|   stm32f401_d_e_uqfn48 IBIS Model
[IBIS ver]   4.2
[File name]  stm32f401_d_e_uqfn48.ibs
[File Rev]   1.0
[Date]   09-06-2015
[Source] Data Created at STMicroelectronics
[Notes]   File originated from ELDO simulations.
[Disclaimer]  This information is for modeling purpose only and is
   not guaranted. The information is subject to change without
   notice.
[Copyright] Copyright 2015 STMicroelectronics Inc.
[Component] stm32f401_d_e_uqfn48
[Manufacturer] STMicroelectronics
[Package]
| variable   typ   min   max
R_pkg   0.0   NA   NA
L_pkg   0.0H   NA   NA
C_pkg   0.0F   NA   NA
[Pin]   signal_name   model_name   R_pin   L_pin   C_pin
1 VBAT POWER 0.053 3.42534E-09 9.041E-14
2 PC13-ANTI_TAMP io8p_arwsudq_ft_v33 0.048377332 2.91404E-09 6.443E-14
3 PC14-OSC32_IN io8p_arwsudq_ft 0.044678997 2.50442E-09 4.365E-14
4 PC15-OSC32_OUT io8p_arsudq_ft 0.041905328 2.19704E-09 2.807E-14
5 PH0-OSC_IN io8p_arsudq_ft 0.040056325 1.9919E-09 1.769E-14
6 PH1-OSC_OUT io8p_arsudq_ft 0.03913 1.89021E-09 1.24625E-14
7 NRST ioreset_ft_v33 0.03913 1.89021E-09 1.24625E-14
8 VSSA GND 0.040057312 1.98992E-09 1.775E-14
9 VDDA POWER 0.041906973 2.19374E-09 2.817E-14
10 PA0-WKUP io8p_arwsudq_ft_v33 0.0446813 2.4998E-09 4.379E-14
11 PA1 io8p_arwsudq_ft 0.048380293 2.9081E-09 6.461E-14
12 PA2 io8p_arwsudq_ft 0.053 3.42534E-09 9.041E-14
13 PA3 io8p_arwsudq_ft 0.053 3.42534E-09 9.041E-14
14 PA4 io8p_ar3wsudq_ft 0.048377332 2.91404E-09 6.443E-14
15 PA5 io8p_ar3wsudq_ft 0.044678997 2.50442E-09 4.365E-14
16 PA6 io8p_ar3wsudq_ft 0.041905328 2.19704E-09 2.807E-14
17 PA7 io8p_arwsudq_ft 0.040056325 1.9919E-09 1.769E-14
18 PB0 io8p_ar3wsudq_ft 0.03913 1.89021E-09 1.24625E-14
19 PB1 io8p_ar3wsudq_ft 0.03913 1.89021E-09 1.24625E-14
20 PB2 io8p_arwsudq_ft 0.040057312 1.98992E-09 1.775E-14
21 PB10 io8p_arsudq_i2cin_ft 0.041906973 2.19374E-09 2.817E-14
22 VCAP1 POWER 0.0446813 2.4998E-09 4.379E-14
23 VSS GND 0.048380293 2.9081E-09 6.461E-14
24 VDD POWER 0.053 3.42534E-09 9.041E-14
25 PB12 io8p_arsudq_ft 0.053 3.42534E-09 9.041E-14
26 PB13 io8p_arsudq_ft 0.048377332 2.91404E-09 6.443E-14
27 PB14 io8p_arsudq_ft 0.044678997 2.50442E-09 4.365E-14
28 PB15 io8p_arsudq_ft 0.041905328 2.19704E-09 2.807E-14
29 PA8 io8p_arsudq_i2cin_ft 0.040056325 1.9919E-09 1.769E-14
30 PA9 io8usb_vbus_otg_ft 0.03913 1.89021E-09 1.24625E-14
31 PA10 io8usb_id_otg_ft 0.03913 1.89021E-09 1.24625E-14
32 PA11 io8usb_lsfs_otg_ft 0.040057312 1.98992E-09 1.775E-14
33 PA12 io8usb_lsfs_otg_ft 0.041906973 2.19374E-09 2.817E-14
34 PA13 io8p_arsudq_ft 0.0446813 2.4998E-09 4.379E-14
35 VSS GND 0.048380293 2.9081E-09 6.461E-14
36 VDD POWER 0.053 3.42534E-09 9.041E-14
37 PA14 io8p_arsudq_ft 0.053 3.42534E-09 9.041E-14
38 PA15 io8p_arsudq_ft 0.048377332 2.91404E-09 6.443E-14
39 PB3 io8p_arsudq_i2cin_ft 0.044678997 2.50442E-09 4.365E-14
40 PB4 io8p_arsudq_i2cin_ft 0.041905328 2.19704E-09 2.807E-14
41 PB5 io8p_ar3wsudq_ft 0.040056325 1.9919E-09 1.769E-14
42 PB6 io8p_arsudq_i2cin_ft 0.03913 1.89021E-09 1.24625E-14
43 PB7 io8p_arsudq_i2cin_ft 0.03913 1.89021E-09 1.24625E-14
44 BOOT0 vpp_test_hv 0.040057312 1.98992E-09 1.775E-14
45 PB8 io8p_arsudq_i2cin_ft 0.041906973 2.19374E-09 2.817E-14
46 PB9 io8p_arsudq_i2cin_ft 0.0446813 2.4998E-09 4.379E-14
47 VSS GND 0.048380293 2.9081E-09 6.461E-14
48 VDD POWER 0.053 3.42534E-09 9.041E-14
[Diff Pin]   inv_pin   vdiff   tdelay_typ  tdelay_min  tdelay_max
32 33 200mV   NA   NA   NA
[Model Selector] io8p_ar3wsudq_ft
io8p00_ar3wsudq_ft_pd_lv  "SPEED00 1P8V, PD=40kOhm"
io8p00_ar3wsudq_ft_pu_lv  "SPEED00 1P8V, PU=40kOhm"
io8p00_ar3wsudq_ft_lv  "SPEED00 1P8V"
io8p01_ar3wsudq_ft_pd_lv  "SPEED01 1P8V, PD=40kOhm"
io8p01_ar3wsudq_ft_pu_lv  "SPEED01 1P8V, PU=40kOhm"
io8p01_ar3wsudq_ft_lv  "SPEED01 1P8V"
io8p10_ar3wsudq_ft_pd_lv  "SPEED10 1P8V, PD=40kOhm"
io8p10_ar3wsudq_ft_pu_lv  "SPEED10 1P8V, PU=40kOhm"
io8p10_ar3wsudq_ft_lv  "SPEED10 1P8V"
io8p11_ar3wsudq_ft_pd_lv  "SPEED11 1P8V, PD=40kOhm"
io8p11_ar3wsudq_ft_pu_lv  "SPEED11 1P8V, PU=40kOhm"
io8p11_ar3wsudq_ft_lv  "SPEED11 1P8V"
io8p00_ar3wsudq_ft_pd  "SPEED00, PD=40kOhm"
io8p00_ar3wsudq_ft_pu  "SPEED00, PU=40kOhm"
io8p00_ar3wsudq_ft  "SPEED00"
io8p01_ar3wsudq_ft_pd  "SPEED01, PD=40kOhm"
io8p01_ar3wsudq_ft_pu  "SPEED01, PU=40kOhm"
io8p01_ar3wsudq_ft  "SPEED01"
io8p10_ar3wsudq_ft_pd  "SPEED10, PD=40kOhm"
io8p10_ar3wsudq_ft_pu  "SPEED10, PU=40kOhm"
io8p10_ar3wsudq_ft  "SPEED10"
io8p11_ar3wsudq_ft_pd  "SPEED11, PD=40kOhm"
io8p11_ar3wsudq_ft_pu  "SPEED11, PU=40kOhm"
io8p11_ar3wsudq_ft  "SPEED11"
[Model Selector] io8p_arsudq_ft
io8p00_arsudq_ft_pd_lv  "SPEED00 1P8V, PD=40kOhm"
io8p00_arsudq_ft_pu_lv  "SPEED00 1P8V, PU=40kOhm"
io8p00_arsudq_ft_lv  "SPEED00 1P8V"
io8p01_arsudq_ft_pd_lv  "SPEED01 1P8V, PD=40kOhm"
io8p01_arsudq_ft_pu_lv  "SPEED01 1P8V, PU=40kOhm"
io8p01_arsudq_ft_lv  "SPEED01 1P8V"
io8p10_arsudq_ft_pd_lv  "SPEED10 1P8V, PD=40kOhm"
io8p10_arsudq_ft_pu_lv  "SPEED10 1P8V, PU=40kOhm"
io8p10_arsudq_ft_lv  "SPEED10 1P8V"
io8p11_arsudq_ft_pd_lv  "SPEED11 1P8V, PD=40kOhm"
io8p11_arsudq_ft_pu_lv  "SPEED11 1P8V, PU=40kOhm"
io8p11_arsudq_ft_lv  "SPEED11 1P8V"
io8p00_arsudq_ft_pd  "SPEED00, PD=40kOhm"
io8p00_arsudq_ft_pu  "SPEED00, PU=40kOhm"
io8p00_arsudq_ft  "SPEED00"
io8p01_arsudq_ft_pd  "SPEED01, PD=40kOhm"
io8p01_arsudq_ft_pu  "SPEED01, PU=40kOhm"
io8p01_arsudq_ft  "SPEED01"
io8p10_arsudq_ft_pd  "SPEED10, PD=40kOhm"
io8p10_arsudq_ft_pu  "SPEED10, PU=40kOhm"
io8p10_arsudq_ft  "SPEED10"
io8p11_arsudq_ft_pd  "SPEED11, PD=40kOhm"
io8p11_arsudq_ft_pu  "SPEED11, PU=40kOhm"
io8p11_arsudq_ft  "SPEED11"
[Model Selector] io8p_arsudq_i2cin_ft
io8p00_arsudq_i2cin_ft_pd_lv  "SPEED00 1P8V, PD=40kOhm"
io8p00_arsudq_i2cin_ft_pu_lv  "SPEED00 1P8V, PU=40kOhm"
io8p00_arsudq_i2cin_ft_lv  "SPEED00 1P8V"
io8p01_arsudq_i2cin_ft_pd_lv  "SPEED01 1P8V, PD=40kOhm"
io8p01_arsudq_i2cin_ft_pu_lv  "SPEED01 1P8V, PU=40kOhm"
io8p01_arsudq_i2cin_ft_lv  "SPEED01 1P8V"
io8p10_arsudq_i2cin_ft_pd_lv  "SPEED10 1P8V, PD=40kOhm"
io8p10_arsudq_i2cin_ft_pu_lv  "SPEED10 1P8V, PU=40kOhm"
io8p10_arsudq_i2cin_ft_lv  "SPEED10 1P8V"
io8p11_arsudq_i2cin_ft_pd_lv  "SPEED11 1P8V, PD=40kOhm"
io8p11_arsudq_i2cin_ft_pu_lv  "SPEED11 1P8V, PU=40kOhm"
io8p11_arsudq_i2cin_ft_lv  "SPEED11 1P8V"
io8p00_arsudq_i2cin_ft_pd  "SPEED00, PD=40kOhm"
io8p00_arsudq_i2cin_ft_pu  "SPEED00, PU=40kOhm"
io8p00_arsudq_i2cin_ft  "SPEED00"
io8p01_arsudq_i2cin_ft_pd  "SPEED01, PD=40kOhm"
io8p01_arsudq_i2cin_ft_pu  "SPEED01, PU=40kOhm"
io8p01_arsudq_i2cin_ft  "SPEED01"
io8p10_arsudq_i2cin_ft_pd  "SPEED10, PD=40kOhm"
io8p10_arsudq_i2cin_ft_pu  "SPEED10, PU=40kOhm"
io8p10_arsudq_i2cin_ft  "SPEED10"
io8p11_arsudq_i2cin_ft_pd  "SPEED11, PD=40kOhm"
io8p11_arsudq_i2cin_ft_pu  "SPEED11, PU=40kOhm"
io8p11_arsudq_i2cin_ft  "SPEED11"
[Model Selector] io8p_arwsudq_ft
io8p00_arwsudq_ft_pd_lv  "SPEED00 1P8V, PD=40kOhm"
io8p00_arwsudq_ft_pu_lv  "SPEED00 1P8V, PU=40kOhm"
io8p00_arwsudq_ft_lv  "SPEED00 1P8V"
io8p01_arwsudq_ft_pd_lv  "SPEED01 1P8V, PD=40kOhm"
io8p01_arwsudq_ft_pu_lv  "SPEED01 1P8V, PU=40kOhm"
io8p01_arwsudq_ft_lv  "SPEED01 1P8V"
io8p10_arwsudq_ft_pd_lv  "SPEED10 1P8V, PD=40kOhm"
io8p10_arwsudq_ft_pu_lv  "SPEED10 1P8V, PU=40kOhm"
io8p10_arwsudq_ft_lv  "SPEED10 1P8V"
io8p11_arwsudq_ft_pd_lv  "SPEED11 1P8V, PD=40kOhm"
io8p11_arwsudq_ft_pu_lv  "SPEED11 1P8V, PU=40kOhm"
io8p11_arwsudq_ft_lv  "SPEED11 1P8V"
io8p00_arwsudq_ft_pd  "SPEED00, PD=40kOhm"
io8p00_arwsudq_ft_pu  "SPEED00, PU=40kOhm"
io8p00_arwsudq_ft  "SPEED00"
io8p01_arwsudq_ft_pd  "SPEED01, PD=40kOhm"
io8p01_arwsudq_ft_pu  "SPEED01, PU=40kOhm"
io8p01_arwsudq_ft  "SPEED01"
io8p10_arwsudq_ft_pd  "SPEED10, PD=40kOhm"
io8p10_arwsudq_ft_pu  "SPEED10, PU=40kOhm"
io8p10_arwsudq_ft  "SPEED10"
io8p11_arwsudq_ft_pd  "SPEED11, PD=40kOhm"
io8p11_arwsudq_ft_pu  "SPEED11, PU=40kOhm"
io8p11_arwsudq_ft  "SPEED11"
[Model Selector] io8p_arwsudq_ft_v33
io8p00_arwsudq_ft_v33_pd_lv  "SPEED00 1P8V, PD=40kOhm"
io8p00_arwsudq_ft_v33_pu_lv  "SPEED00 1P8V, PU=40kOhm"
io8p00_arwsudq_ft_v33_lv  "SPEED00 1P8V"
io8p01_arwsudq_ft_v33_pd_lv  "SPEED01 1P8V, PD=40kOhm"
io8p01_arwsudq_ft_v33_pu_lv  "SPEED01 1P8V, PU=40kOhm"
io8p01_arwsudq_ft_v33_lv  "SPEED01 1P8V"
io8p10_arwsudq_ft_v33_pd_lv  "SPEED10 1P8V, PD=40kOhm"
io8p10_arwsudq_ft_v33_pu_lv  "SPEED10 1P8V, PU=40kOhm"
io8p10_arwsudq_ft_v33_lv  "SPEED10 1P8V"
io8p11_arwsudq_ft_v33_pd_lv  "SPEED11 1P8V, PD=40kOhm"
io8p11_arwsudq_ft_v33_pu_lv  "SPEED11 1P8V, PU=40kOhm"
io8p11_arwsudq_ft_v33_lv  "SPEED11 1P8V"
io8p00_arwsudq_ft_v33_pd  "SPEED00, PD=40kOhm"
io8p00_arwsudq_ft_v33_pu  "SPEED00, PU=40kOhm"
io8p00_arwsudq_ft_v33  "SPEED00"
io8p01_arwsudq_ft_v33_pd  "SPEED01, PD=40kOhm"
io8p01_arwsudq_ft_v33_pu  "SPEED01, PU=40kOhm"
io8p01_arwsudq_ft_v33  "SPEED01"
io8p10_arwsudq_ft_v33_pd  "SPEED10, PD=40kOhm"
io8p10_arwsudq_ft_v33_pu  "SPEED10, PU=40kOhm"
io8p10_arwsudq_ft_v33  "SPEED10"
io8p11_arwsudq_ft_v33_pd  "SPEED11, PD=40kOhm"
io8p11_arwsudq_ft_v33_pu  "SPEED11, PU=40kOhm"
io8p11_arwsudq_ft_v33  "SPEED11"
[Model Selector] io8usb_id_otg_ft
io8p00_id_otg_ft_pd_lv  "SPEED00 1P8V, PD=14kOhm"
io8p00_id_otg_ft_pu_lv  "SPEED00 1P8V, PU=14kOhm"
io8p00_id_otg_ft_lv  "SPEED00 1P8V"
io8p01_id_otg_ft_pd_lv  "SPEED01 1P8V, PD=14kOhm"
io8p01_id_otg_ft_pu_lv  "SPEED01 1P8V, PU=14kOhm"
io8p01_id_otg_ft_lv  "SPEED01 1P8V"
io8p10_id_otg_ft_pd_lv  "SPEED10 1P8V, PD=14kOhm"
io8p10_id_otg_ft_pu_lv  "SPEED10 1P8V, PU=14kOhm"
io8p10_id_otg_ft_lv  "SPEED10 1P8V"
io8p11_id_otg_ft_pd_lv  "SPEED11 1P8V, PD=14kOhm"
io8p11_id_otg_ft_pu_lv  "SPEED11 1P8V, PU=14kOhm"
io8p11_id_otg_ft_lv  "SPEED11 1P8V"
io8p00_id_otg_ft_pd  "SPEED00, PD=14kOhm"
io8p00_id_otg_ft_pu  "SPEED00, PU=14kOhm"
io8p00_id_otg_ft  "SPEED00"
io8p01_id_otg_ft_pd  "SPEED01, PD=14kOhm"
io8p01_id_otg_ft_pu  "SPEED01, PU=14kOhm"
io8p01_id_otg_ft  "SPEED01"
io8p10_id_otg_ft_pd  "SPEED10, PD=14kOhm"
io8p10_id_otg_ft_pu  "SPEED10, PU=14kOhm"
io8p10_id_otg_ft  "SPEED10"
io8p11_id_otg_ft_pd  "SPEED11, PD=14kOhm"
io8p11_id_otg_ft_pu  "SPEED11, PU=14kOhm"
io8p11_id_otg_ft  "SPEED11"
[Model Selector] io8usb_lsfs_otg_ft
io8usb_ls_otg_ft_dpdn_pd  "LS USB DP/DN IO + PD=20kOhm"
io8usb_ls_otg_ft_dpdn_pupu2  "LS USB DP/DN IO + PU/PU2=2.2kOhm"
io8usb_ls_otg_ft_dpdn_pu2  "LS USB DP/DN IO + PU2=1.2kOhm"
io8usb_ls_otg_ft_dpdn_pu  "LS USB DP/DN IO + PU=1.2kOhm"
io8usb_ls_otg_ft_dpdn  "LS USB DP/DN IO"
io8usb_fs_otg_ft_dpdn_pd  "HS USB DP/DN IO + PD=20kOhm"
io8usb_fs_otg_ft_dpdn_pupu2  "HS USB DP/DN IO + PU/PU2=2.2kOhm"
io8usb_fs_otg_ft_dpdn_pu2  "HS USB DP/DN IO + PU2=1.2kOhm"
io8usb_fs_otg_ft_dpdn_pu  "HS USB DP/DN IO + PU=1.2kOhm"
io8usb_fs_otg_ft_dpdn  "HS USB DP/DN IO"
io8p00_lsfs_otg_ft_pd_lv  "SPEED00 1P8V, PD=40kOhm"
io8p00_lsfs_otg_ft_pu_lv  "SPEED00 1P8V, PU=40kOhm"
io8p00_lsfs_otg_ft_lv  "SPEED00 1P8V"
io8p01_lsfs_otg_ft_pd_lv  "SPEED01 1P8V, PD=40kOhm"
io8p01_lsfs_otg_ft_pu_lv  "SPEED01 1P8V, PU=40kOhm"
io8p01_lsfs_otg_ft_lv  "SPEED01 1P8V"
io8p10_lsfs_otg_ft_pd_lv  "SPEED10 1P8V, PD=40kOhm"
io8p10_lsfs_otg_ft_pu_lv  "SPEED10 1P8V, PU=40kOhm"
io8p10_lsfs_otg_ft_lv  "SPEED10 1P8V"
io8p11_lsfs_otg_ft_pd_lv  "SPEED11 1P8V, PD=40kOhm"
io8p11_lsfs_otg_ft_pu_lv  "SPEED11 1P8V, PU=40kOhm"
io8p11_lsfs_otg_ft_lv  "SPEED11 1P8V"
io8p00_lsfs_otg_ft_pd  "SPEED00, PD=40kOhm"
io8p00_lsfs_otg_ft_pu  "SPEED00, PU=40kOhm"
io8p00_lsfs_otg_ft  "SPEED00"
io8p01_lsfs_otg_ft_pd  "SPEED01, PD=40kOhm"
io8p01_lsfs_otg_ft_pu  "SPEED01, PU=40kOhm"
io8p01_lsfs_otg_ft  "SPEED01"
io8p10_lsfs_otg_ft_pd  "SPEED10, PD=40kOhm"
io8p10_lsfs_otg_ft_pu  "SPEED10, PU=40kOhm"
io8p10_lsfs_otg_ft  "SPEED10"
io8p11_lsfs_otg_ft_pd  "SPEED11, PD=40kOhm"
io8p11_lsfs_otg_ft_pu  "SPEED11, PU=40kOhm"
io8p11_lsfs_otg_ft  "SPEED11"
[Model Selector] io8usb_vbus_otg_ft
io8psenb_vbus_otg_ft  "VBUS PULSE, SENSE VB"
io8psenab_vbus_otg_ft  "VBUS PULSE, SENSE VA and VB"
io8psena_vbus_otg_ft  "VBUS PULSE, SENSE VA"
io8psen_vbus_otg_ft  "VBUS PULSE"
io8p00_vbus_otg_ft_pd_lv  "SPEED00 1P8V, PD=40kOhm"
io8p00_vbus_otg_ft_pu_lv  "SPEED00 1P8V, PU=40kOhm"
io8p00_vbus_otg_ft_lv  "SPEED00 1P8V"
io8p01_vbus_otg_ft_pd_lv  "SPEED01 1P8V, PD=40kOhm"
io8p01_vbus_otg_ft_pu_lv  "SPEED01 1P8V, PU=40kOhm"
io8p01_vbus_otg_ft_lv  "SPEED01 1P8V"
io8p10_vbus_otg_ft_pd_lv  "SPEED10 1P8V, PD=40kOhm"
io8p10_vbus_otg_ft_pu_lv  "SPEED10 1P8V, PU=40kOhm"
io8p10_vbus_otg_ft_lv  "SPEED10 1P8V"
io8p11_vbus_otg_ft_pd_lv  "SPEED11 1P8V, PD=40kOhm"
io8p11_vbus_otg_ft_pu_lv  "SPEED11 1P8V, PU=40kOhm"
io8p11_vbus_otg_ft_lv  "SPEED11 1P8V"
io8p00_vbus_otg_ft_pd  "SPEED00, PD=40kOhm"
io8p00_vbus_otg_ft_pu  "SPEED00, PU=40kOhm"
io8p00_vbus_otg_ft  "SPEED00"
io8p01_vbus_otg_ft_pd  "SPEED01, PD=40kOhm"
io8p01_vbus_otg_ft_pu  "SPEED01, PU=40kOhm"
io8p01_vbus_otg_ft  "SPEED01"
io8p10_vbus_otg_ft_pd  "SPEED10, PD=40kOhm"
io8p10_vbus_otg_ft_pu  "SPEED10, PU=40kOhm"
io8p10_vbus_otg_ft  "SPEED10"
io8p11_vbus_otg_ft_pd  "SPEED11, PD=40kOhm"
io8p11_vbus_otg_ft_pu  "SPEED11, PU=40kOhm"
io8p11_vbus_otg_ft  "SPEED11"
[Model Selector] ioreset_ft_v33
ioreset_ft_v33_pu_lv  "ioreset 1P8V + PU=40kOhm"
ioreset_ft_v33_nopu_lv  "ioreset 1P8V"
ioreset_ft_v33_pu  "ioreset + PU=40kOhm"
ioreset_ft_v33_nopu  "ioreset"
[Model Selector] vpp_test_hv
vpp_test_hv_2p4  "Input Buffer 1P8V"
vpp_test_hv_3p3  "Input Buffer"
| Models and submodels in the file (212): io8p00_ar3wsudq_ft_pd_lv (I/O), io8p00_ar3wsudq_ft_pu_lv (I/O), io8p00_ar3wsudq_ft_lv (I/O), io8p01_ar3wsudq_ft_pd_lv (I/O), io8p01_ar3wsudq_ft_pu_lv (I/O), io8p01_ar3wsudq_ft_lv (I/O), io8p10_ar3wsudq_ft_pd_lv (I/O), io8p10_ar3wsudq_ft_pu_lv (I/O), io8p10_ar3wsudq_ft_lv (I/O), io8p11_ar3wsudq_ft_pd_lv (I/O), io8p11_ar3wsudq_ft_pu_lv (I/O), io8p11_ar3wsudq_ft_lv (I/O), io8p00_ar3wsudq_ft_pd (I/O), io8p00_ar3wsudq_ft_pu (I/O), io8p00_ar3wsudq_ft (I/O), io8p01_ar3wsudq_ft_pd (I/O), io8p01_ar3wsudq_ft_pu (I/O), io8p01_ar3wsudq_ft (I/O), io8p10_ar3wsudq_ft_pd (I/O), io8p10_ar3wsudq_ft_pu (I/O), io8p10_ar3wsudq_ft (I/O), io8p11_ar3wsudq_ft_pd (I/O), io8p11_ar3wsudq_ft_pu (I/O), io8p11_ar3wsudq_ft (I/O), io8p00_arsudq_ft_pd_lv (I/O), io8p00_arsudq_ft_pu_lv (I/O), io8p00_arsudq_ft_lv (I/O), io8p01_arsudq_ft_pd_lv (I/O), io8p01_arsudq_ft_pu_lv (I/O), io8p01_arsudq_ft_lv (I/O), io8p10_arsudq_ft_pd_lv (I/O), io8p10_arsudq_ft_pu_lv (I/O), io8p10_arsudq_ft_lv (I/O), io8p11_arsudq_ft_pd_lv (I/O), io8p11_arsudq_ft_pu_lv (I/O), io8p11_arsudq_ft_lv (I/O), io8p00_arsudq_ft_pd (I/O), io8p00_arsudq_ft_pu (I/O), io8p00_arsudq_ft (I/O), io8p01_arsudq_ft_pd (I/O), io8p01_arsudq_ft_pu (I/O), io8p01_arsudq_ft (I/O), io8p10_arsudq_ft_pd (I/O), io8p10_arsudq_ft_pu (I/O), io8p10_arsudq_ft (I/O), io8p11_arsudq_ft_pd (I/O), io8p11_arsudq_ft_pu (I/O), io8p11_arsudq_ft (I/O), io8p00_arsudq_i2cin_ft_pd_lv (I/O), io8p00_arsudq_i2cin_ft_pu_lv (I/O), io8p00_arsudq_i2cin_ft_lv (I/O), io8p01_arsudq_i2cin_ft_pd_lv (I/O), io8p01_arsudq_i2cin_ft_pu_lv (I/O), io8p01_arsudq_i2cin_ft_lv (I/O), io8p10_arsudq_i2cin_ft_pd_lv (I/O), io8p10_arsudq_i2cin_ft_pu_lv (I/O), io8p10_arsudq_i2cin_ft_lv (I/O), io8p11_arsudq_i2cin_ft_pd_lv (I/O), io8p11_arsudq_i2cin_ft_pu_lv (I/O), io8p11_arsudq_i2cin_ft_lv (I/O), io8p00_arsudq_i2cin_ft_pd (I/O), io8p00_arsudq_i2cin_ft_pu (I/O), io8p00_arsudq_i2cin_ft (I/O), io8p01_arsudq_i2cin_ft_pd (I/O), io8p01_arsudq_i2cin_ft_pu (I/O), io8p01_arsudq_i2cin_ft (I/O), io8p10_arsudq_i2cin_ft_pd (I/O), io8p10_arsudq_i2cin_ft_pu (I/O), io8p10_arsudq_i2cin_ft (I/O), io8p11_arsudq_i2cin_ft_pd (I/O), io8p11_arsudq_i2cin_ft_pu (I/O), io8p11_arsudq_i2cin_ft (I/O), io8p00_arwsudq_ft_pd_lv (I/O), io8p00_arwsudq_ft_pu_lv (I/O), io8p00_arwsudq_ft_lv (I/O), io8p01_arwsudq_ft_pd_lv (I/O), io8p01_arwsudq_ft_pu_lv (I/O), io8p01_arwsudq_ft_lv (I/O), io8p10_arwsudq_ft_pd_lv (I/O), io8p10_arwsudq_ft_pu_lv (I/O)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
